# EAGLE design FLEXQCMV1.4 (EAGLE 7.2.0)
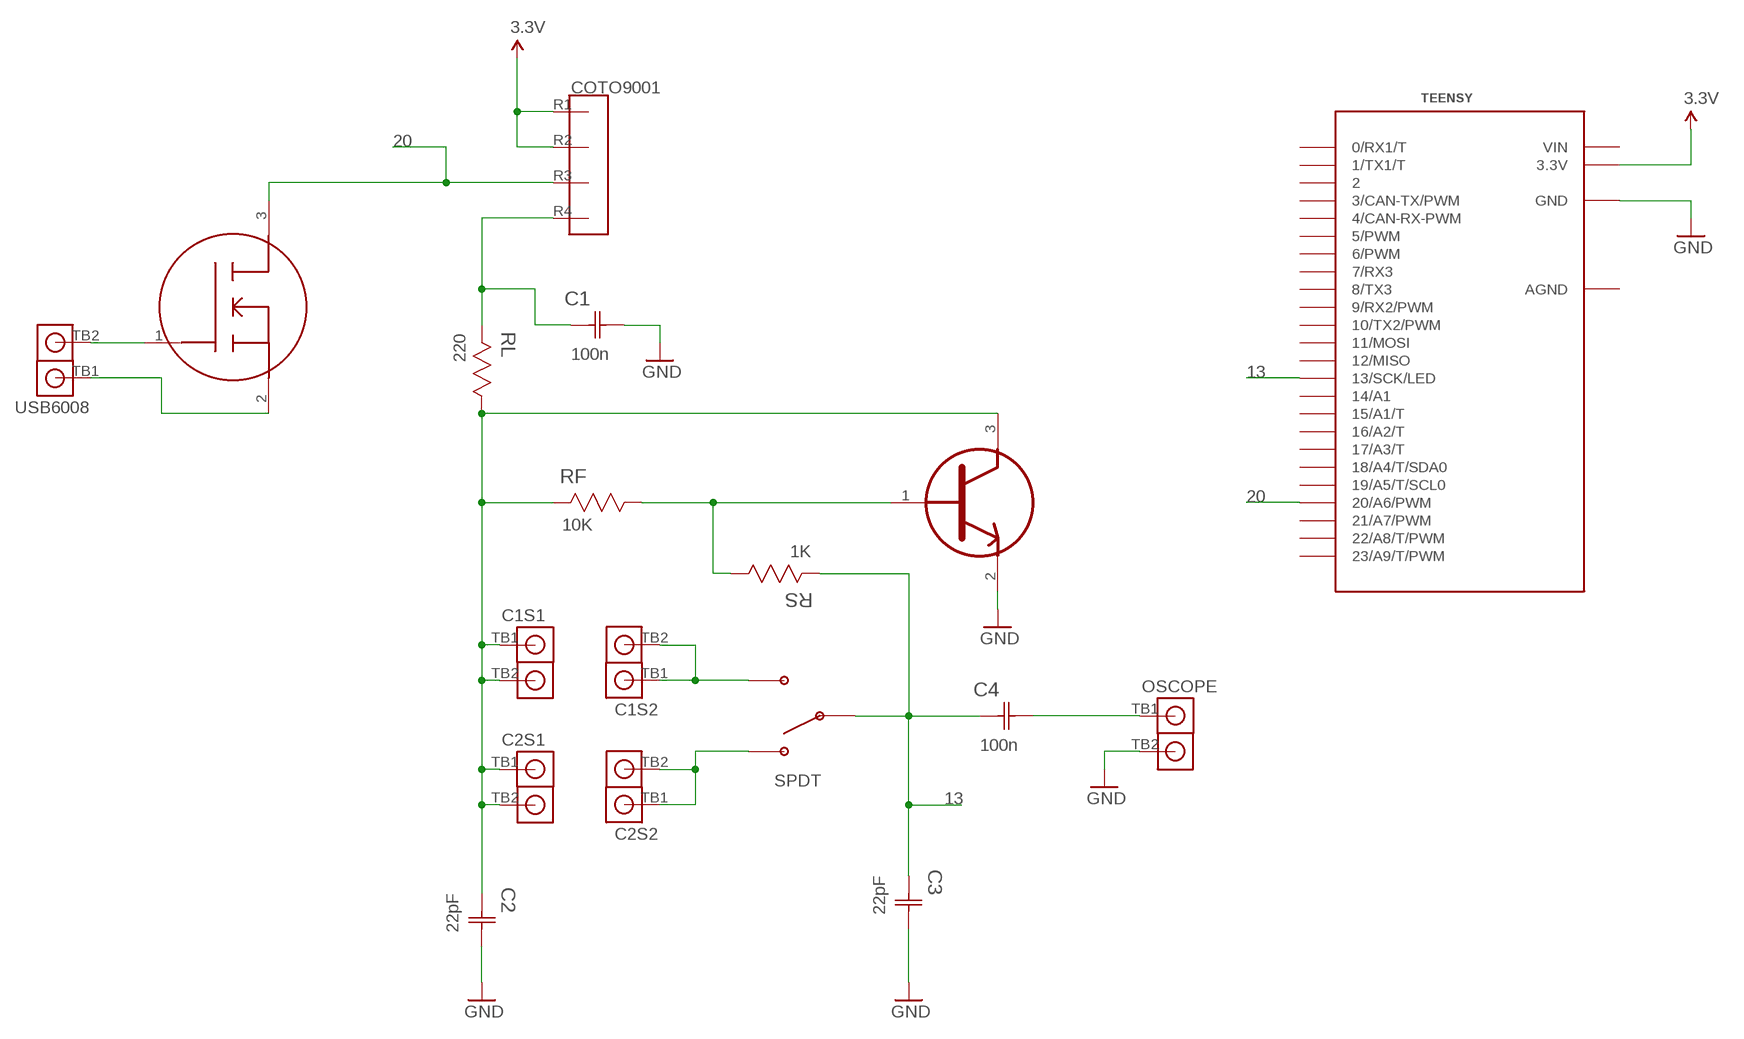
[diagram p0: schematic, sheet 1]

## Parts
C1  100n  C1206C104K1RACTU  [CAPC3216X88N]
C1S1  TERMBLOCKX2  [TERMBLOCKX2]
C1S2  TERMBLOCKX2  [TERMBLOCKX2]
C2  22pF  C1206C220J5GACTU  [CAPC3216X88N]
C2S1  TERMBLOCKX2  [TERMBLOCKX2]
C2S2  TERMBLOCKX2  [TERMBLOCKX2]
C3  22pF  C1206C220J5GACTU  [CAPC3216X88N]
C4  100n  C1206C104K1RACTU  [CAPC3216X88N]
COTO9001  COTO9001  [COTO9001]
OSCOPE  TERMBLOCKX2  [TERMBLOCKX2]
RF  10K  CRCW120610K0FKEA  [RESC3216X71N]
RL  220  CRCW1206220RJNEA  [RESC3216X71N]
RS  1K  CRCW12061K00FKEA  [RESC3216X71N]
SPDT  SPDTSWITCH  [SPDTSWITCH]
TEENSY  TEENSY_3.1_DIL  [TEENSY3-DIL]
U1  FET  2N7002K  [SOT95P230X110-3N]
U2  BJT  BC847C  [SOT95P230X110-3N]
USB6008  TERMBLOCKX2  [TERMBLOCKX2]

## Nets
3.3V: COTO9001.R1 COTO9001.R2 TEENSY.3.3V
13: C3.1(C1) C4.1(C1) RS.2 SPDT.SW2 TEENSY.13(13/SCK/LED)
20: COTO9001.R3 TEENSY.20/A6(20/A6/PWM) U1.3(D)
GND: C1.2(C2) C2.2(C2) C3.2(C2) OSCOPE.TB2 TEENSY.GND U2.2(E)
N$1: U1.1(G) USB6008.TB2
N$2: U1.2(S) USB6008.TB1
N$3: C1.1(C1) COTO9001.R4 RL.2
N$4: C1S2.TB1 C1S2.TB2 SPDT.SW3
N$5: RF.1 RS.1 U2.1(B)
N$6: C2S2.TB1 C2S2.TB2 SPDT.SW1
N$7: C1S1.TB1 C1S1.TB2 C2.1(C1) C2S1.TB1 C2S1.TB2 RF.2 RL.1 U2.3(C)
N$8: C4.2(C2) OSCOPE.TB1
Unconnected: TEENSY.0(0/RX1/T) TEENSY.1(1/TX1/T) TEENSY.2 TEENSY.3(3/CAN-TX/PWM) TEENSY.4(4/CAN-RX-PWM) TEENSY.5(5/PWM) TEENSY.6(6/PWM) TEENSY.7(7/RX3) TEENSY.8(8/TX3) TEENSY.9(9/RX2/PWM) TEENSY.10(10/TX2/PWM) TEENSY.11(11/MOSI) TEENSY.12(12/MISO) TEENSY.14/A0(14/A1) TEENSY.15/A1(15/A1/T) TEENSY.16/A2(16/A2/T) TEENSY.17/A3(17/A3/T) TEENSY.18/A4(18/A4/T/SDA0) TEENSY.19/A5(19/A5/T/SCL0) TEENSY.21/A7(21/A7/PWM) TEENSY.22/A8(22/A8/T/PWM) TEENSY.23/A9(23/A9/T/PWM)

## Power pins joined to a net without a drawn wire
AGND: TEENSY.AGND
VIN: TEENSY.VIN

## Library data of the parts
C1 C4 = Kemet_By_element14_Batch_1:C1206C104K1RACTU: CAPACITOR, 1206; MPN: C1206C104K1RACTU; OC_FARNELL: 1414714; OC_NEWARK: 85C2205; SUPPLIER: Kemet; TOLERANCE: ±10%; VALUE: 100nF; VOLTAGERATING: 100V
C1S1 C1S2 C2S1 C2S2 OSCOPE USB6008 = FLEXQCMLIBRARY:TERMBLOCKX2
C2 C3 = Kemet_By_element14_Batch_1:C1206C220J5GACTU: CAPACITOR, 1206; MPN: C1206C220J5GACTU; OC_FARNELL: 1414717; OC_NEWARK: 70K9304; SUPPLIER: Kemet; TOLERANCE: ±5%; VOLTAGERATING: 50V
COTO9001 = FLEXQCMLIBRARY:COTO9001
RF = Vishay_By_element14_Batch_1:CRCW120610K0FKEA: RESISTOR, 1206; MPN: CRCW120610K0FKEA; OC_FARNELL: 1469970; OC_NEWARK: 53K1907; SUPPLIER: Vishay; TOLERANCE: ±1%; VALUE: 10K Ohms; WATTAGE: 0.25W
RL = Vishay_By_element14_Batch_1:CRCW1206220RJNEA: RESISTOR, 1206; MPN: CRCW1206220RJNEA; OC_FARNELL: -; OC_NEWARK: 59M6970; SUPPLIER: Vishay; TOLERANCE: ±5%; VALUE: 220 Ohms; WATTAGE: 0.25W
RS = Vishay_By_element14_Batch_1:CRCW12061K00FKEA: RESISTOR, 1206; MPN: CRCW12061K00FKEA; OC_FARNELL: 1469965; OC_NEWARK: 53K1780; SUPPLIER: Vishay; TOLERANCE: ±1%; VALUE: 1K Ohms; WATTAGE: 0.25W
SPDT = FLEXQCMLIBRARY:SPDTSWITCH
TEENSY = Teensy_3_and_LC_Series_Boards_v1.0:TEENSY_3.1_DIL: Teensy 3.1 or 3.2 in a DIL Layout.
U1 = NXP_By_element14_Batch_1:2N7002K: logic level FET; MPN: 2N7002K; OC_FARNELL: 1758065; OC_NEWARK: -; PACKAGE: SOT-3; SUPPLIER: NXP Semiconductors
U2 = NXP_By_element14_Batch_1:BC847C

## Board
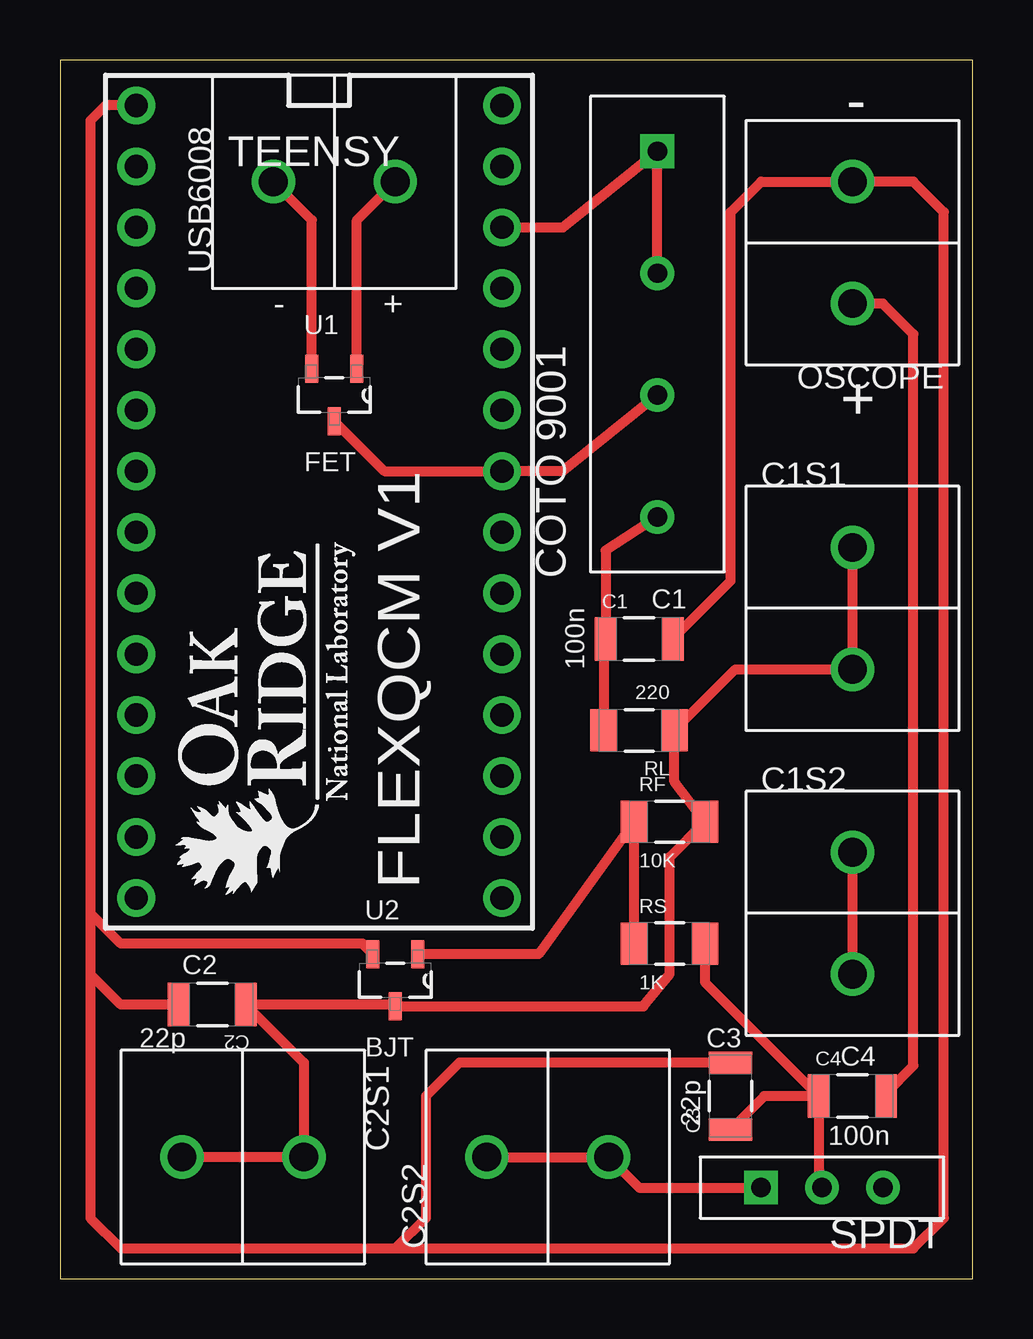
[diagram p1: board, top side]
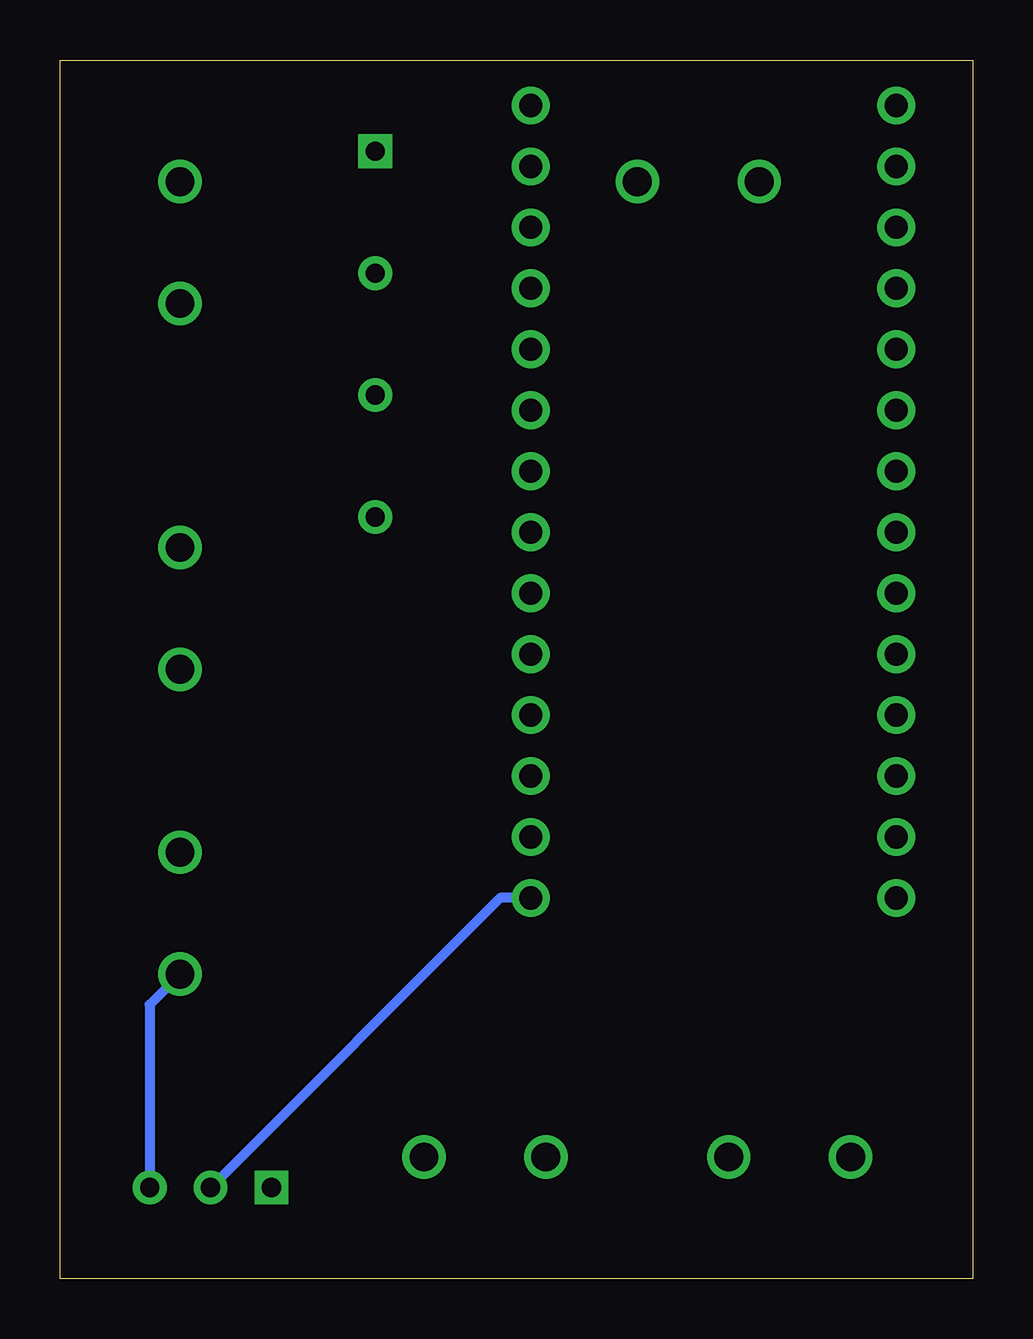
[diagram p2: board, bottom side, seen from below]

Size 38.02 x 50.79 mm. Coordinates in mm from the lower left corner, seen from the top.
Outline: 0,0 38.02,0 38.02,50.79 0,50.79 0,0
Copper layers (1*16): Top 0.035mm / dielectric 1.5mm / Bottom 0.035mm
Design rules "SparkFun": minimum track width 8mil, minimum drill 20mil, track to track 8mil, track to pad 8mil, pad to pad 8mil, via to via 8mil, smd to smd 8mil, copper to edge 10mil, drill to drill 8mil, minimum pad ring 12mil, minimum via ring 10mil, stop-mask expansion 4mil, vias tented up to drill 25mil, thermal gap 10mil

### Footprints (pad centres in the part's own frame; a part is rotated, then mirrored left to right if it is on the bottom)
CAPC3216X88N = smd 0.914 x 1.803: 1 -1.397,0; 2 1.397,0
TERMBLOCKX2 = drill 1.2: TB1 0,2.54; TB2 0,-2.54
COTO9001 = drill 0.8 square: R1 0,7.62 | drill 0.8: R2 0,2.54; R3 0,-2.54; R4 0,-7.62
RESC3216X71N = smd 1.118 x 1.753: 1 -1.473,0; 2 1.473,0
SPDTSWITCH = drill 0.8 square: SW1 0,2.54 | drill 0.8: SW2 0,0; SW3 0,-2.54
TEENSY3-DIL = drill 0.965: 0 -7.62,13.97; 1 -7.62,11.43; 2 -7.62,8.89; 3 -7.62,6.35; 3.3V 7.62,11.43; 4 -7.62,3.81; 5 -7.62,1.27; 6 -7.62,-1.27; 7 -7.62,-3.81; 8 -7.62,-6.35; 9 -7.62,-8.89; 10 -7.62,-11.43; 11 -7.62,-13.97; 12 -7.62,-16.51; 13 7.62,-16.51; 14/A0 7.62,-13.97; 15/A1 7.62,-11.43; 16/A2 7.62,-8.89; 17/A3 7.62,-6.35; 18/A4 7.62,-3.81; 19/A5 7.62,-1.27; 20/A6 7.62,1.27; 21/A7 7.62,3.81; 22/A8 7.62,6.35; 23/A9 7.62,8.89; AGND 7.62,13.97; GND -7.62,16.51; VIN 7.62,16.51
SOT95P230X110-3N = smd 1.168 x 0.533: 1 -1.092,0.94; 2 -1.092,-0.94; 3 1.092,0

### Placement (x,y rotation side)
C1  24.13,26.67 0 top
C1S1  33.02,27.94 0 top
C1S2  33.02,15.24 0 top
C2  6.35,11.43 180 top
C2S1  7.62,5.08 270 top
C2S2  20.32,5.08 90 top
C3  27.94,7.62 90 top
C4  33.02,7.62 0 top
COTO9001  24.89,39.37 0 top
OSCOPE  33.02,43.18 180 top
RF  25.4,19.05 0 top
RL  24.13,22.86 180 top
RS  25.4,13.97 0 top
SPDT  31.75,3.81 90 top
TEENSY  10.79,32.38 0 top
U1  11.43,36.83 270 top
U2  13.97,12.45 270 top
U$1  [ORNLLOGOV9]  12.45,15.75 90 top
USB6008  11.43,45.72 90 top

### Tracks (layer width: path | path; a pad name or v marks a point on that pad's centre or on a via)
3.3V
  Top 0.406: TEENSY.3.3V 20.95,43.81 COTO9001.R1 COTO9001.R2
13
  Top 0.406: C4.1 31.62,3.94 SPDT.SW2 | C4.1 29.34,7.62 C3.1 | RS.2 26.87,12.37 C4.1
  Bottom 0.406: TEENSY.13 19.68,15.88 SPDT.SW2
20
  Top 0.406: U1.3 13.51,33.66 TEENSY.20/A6 20.95,33.66 COTO9001.R3
GND
  Top 0.406: TEENSY.GND 1.91,48.9 1.27,48.26 1.27,15.24 | 1.27,15.24 1.27,12.7 | 1.27,12.7 1.27,2.54 2.54,1.27 13.97,1.27 | 13.97,1.27 35.56,1.27 36.83,2.54 36.83,44.45 35.56,45.72 OSCOPE.TB2 29.21,45.72 27.94,44.45 27.94,29.08 C1.2 | C2.2 2.54,11.43 1.27,12.7 | C3.2 16.64,9.02 15.24,7.62 15.24,2.54 13.97,1.27 | U2.2 12.6,13.97 2.54,13.97 1.27,15.24
N$1
  Top 0.406: U1.1 12.37,44.12 USB6008.TB2
N$2
  Top 0.406: U1.2 10.49,44.12 USB6008.TB1
N$3
  Top 0.406: COTO9001.R4 22.73,30.35 C1.1 22.66,26.59 RL.2
N$4
  Top 0.406: C1S2.TB1 C1S2.TB2
  Bottom 0.406: C1S2.TB2 34.29,11.43 SPDT.SW3
N$5
  Top 0.406: U2.1 19.94,13.54 RF.1 RS.1
N$6
  Top 0.406: C2S2.TB1 C2S2.TB2 24.13,3.81 SPDT.SW1
N$7
  Top 0.406: C1S1.TB1 C1S1.TB2 28.14,25.4 RL.1 25.6,20.73 RF.2 25.4,17.58 25.4,12.7 24.31,11.35 U2.3 13.89,11.43 C2.1 10.16,9.02 C2S1.TB1 C2S1.TB2
N$8
  Top 0.406: C4.2 34.42,7.75 35.56,8.89 35.56,39.37 34.29,40.64 OSCOPE.TB1

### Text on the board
tPlace: - | - | + | + | C1 | 100n | FLEXQCM V1 | C2 | 22p | C3 | C4 | 22p | 100n

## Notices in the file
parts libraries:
SparkFun-Aesthetics: Licensing: Creative Commons ShareAlike 4.0 International - https://creativecommons.org/licenses/by-sa/4.0
